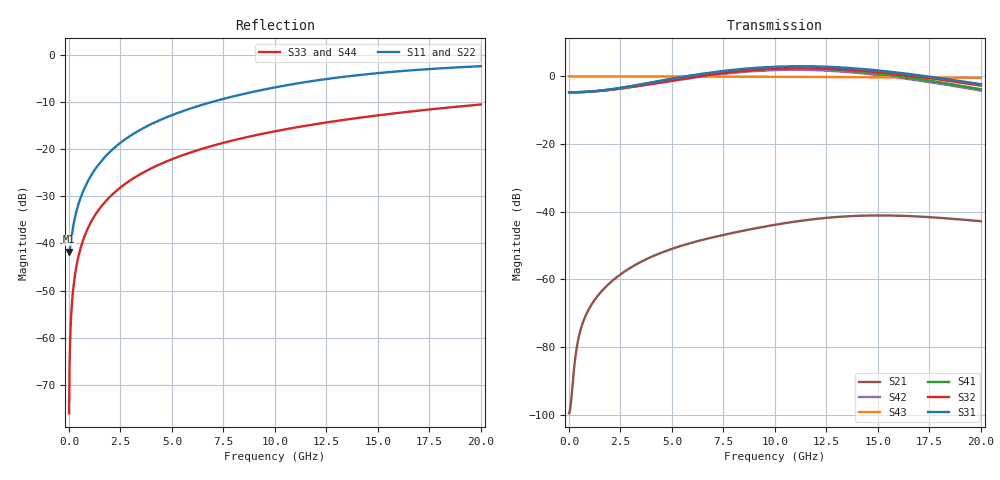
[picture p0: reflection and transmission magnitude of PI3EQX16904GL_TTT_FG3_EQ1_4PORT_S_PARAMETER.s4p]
! NPort=4 DATA=2000 NOISE=0 GROUPDELAY=0 COMPLEX_DATAFORMAT=POLAR
! NumOfBlock=1 NumOfParam=0
! .MODEL Smodel S TSTONEFILE=PI3EQX16904GL_TTT_FG3_EQ1_4PORT_S_PARAMETER.s4p TYPE=S
!  -- The above .MODEL line can be used for the S element in the netlist.
! The s parameter is extracted from the linear redriver, it is not bi-directional; only s(4,1)s(4,2) and s(3,1)s(3,2)
! should be the insertion loss
!Port definition:
!Port1 = input+
!Port2 = input-
!Port3 = output+
!Port4 = output-
# Hz S MA R  50
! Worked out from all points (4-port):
!   2000 points, 10 MHz to 20 GHz, reference 50 ohm
!   strongest paths, dB at 10 MHz, 5.01 GHz, 10.01 GHz, 15.01 GHz, 20 GHz:
!     S31: -4.7, -0.7, 2.9, 1.8, -2.3
!     S32: -4.7, -1.2, 2.3, 1.3, -2.7
!     S41: -4.7, -0.8, 2.4, 0.9, -3.8
!     S43: 0.0, 0.0, -0.1, -0.3, -0.4
!     S42: -4.7, -1.3, 1.9, 0.4, -4.2
!     S21: -99.6, -51.0, -43.9, -41.1, -42.8
!   lowest |S11| = -41.7 dB at 10 MHz (marker M1), VSWR 1.02, Z = 49.2 - j0.0603 ohm
!   |S11| at or under -10 dB: start of sweep to 6.915 GHz
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1e7  0.008182 -175.7  1.049e-05 7.4  0 0.0  0 0.0
     1.049e-05 7.4  0.008182 -175.7  0 0.0  0 0.0
     0.5833 -0.1  0.5833 179.9  0.0001571 -90.0  1 -0.0
     0.5833 179.9  0.5833 -0.1  1 -0.0  0.0001571 -90.0
4e8  0.02342 -118.9  0.0001066 116.6  0 0.0  0 0.0
     0.0001066 116.6  0.02342 -118.9  0 0.0  0 0.0
     0.5842 -0.7  0.5836 178.9  0.006283 -90.4  1 -0.4
     0.5841 178.6  0.5836 -1.8  1 -0.4  0.006283 -90.4
1.68e9  0.07972 -102.7  0.0007173 102.2  0 0.0  0 0.0
        0.0007175 102.2  0.07972 -102.7  0 0.0  0 0.0
        0.6243 -3.2  0.6174 175.2  0.02638 -91.6  0.9996 -1.5
        0.6234 173.8  0.6165 -7.8  0.9996 -1.5  0.02638 -91.6
6.25e9  0.2862 -105.7  0.00369 69.5  0 0.0  0 0.0
        0.00368 69.2  0.2862 -105.8  0 0.0  0 0.0
        1.071 -40.6  0.9949 138.3  0.09767 -95.8  0.9948 -5.6
        1.05 128.3  0.9755 -52.8  0.9948 -5.6  0.09767 -95.8
1.021e10  0.4623 -113.5  0.006616 40.5  0 0.0  0 0.0
          0.006571 40.5  0.4613 -113.6  0 0.0  0 0.0
          1.398 -99.7  1.308 80.7  0.1582 -99.5  0.9864 -9.1
          1.329 62.5  1.243 -117.0  0.9864 -9.1  0.1582 -99.5
1.428e10  0.6193 -123.3  0.00878 3.0  0 0.0  0 0.0
          0.008756 3.2  0.6175 -123.3  0 0.0  0 0.0
          1.285 -166.1  1.214 14.8  0.2184 -103.1  0.9739 -12.6
          1.169 -10.2  1.104 170.7  0.9739 -12.6  0.2184 -103.1
2e10  0.7618 -135.5  0.007294 -38.7  0 0.0  0 0.0
      0.007237 -38.9  0.7603 -135.4  0 0.0  0 0.0
      0.7668 114.0  0.7313 -64.9  0.2986 -108.1  0.9506 -17.4
      0.6456 -97.9  0.6157 83.1  0.9506 -17.4  0.2986 -108.1
